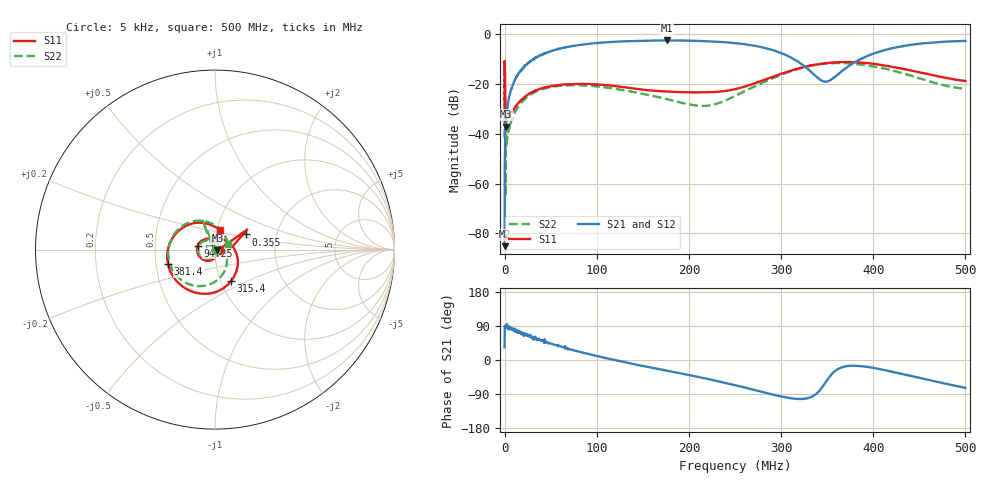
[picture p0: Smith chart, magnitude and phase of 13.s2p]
#  HZ  S  MA  R  50.00
! Rohde & Schwarz Vector Network Analyzer
! Rohde-Schwarz,ZNL6-2Port,1323001206101378,1.50.1.34-21.10.1.104
! Created: UTC 10/21/2024, 2:43:58 AM
! freq[Hz]  mag:S11  ang:S11  mag:S21  ang:S21  mag:S12  ang:S12  mag:S22  ang:S22
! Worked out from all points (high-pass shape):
!   10001 points, 5 kHz to 500 MHz, reference 50 ohm
!   highest |S21| = -2.50 dB at 176.2 MHz (marker M1); lowest = -85.2 dB at 5 kHz (marker M2)
!   |S21| within 3 dB of the highest: 62.95 MHz to 282.4 MHz (219.4 MHz wide, 127 % of centre); 422 MHz to end of sweep
!   lowest |S11| = -37.1 dB at 1.205 MHz (marker M3), VSWR 1.03, Z = 51.3 - j0.451 ohm
!   |S11| at or under -10 dB: start of sweep to end of sweep
!   |S22| runs from -65.2 to -10.9 dB; largest |S21 - S12| = 0.085
!   S11 on the Smith chart (normalised r, x): 5 kHz: 1.05, +0.00; 355 kHz: 1.39, +0.24; 94.25 MHz: 0.82, +0.04; 315.4 MHz: 1.12, -0.41; 381.4 MHz: 0.58, -0.10; 500 MHz: 1.03, +0.23
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5000  0.02251 1.1  5.509e-05 33.7  1.001e-05 114.1  0.008225 -27.2
354996.5  0.1909 26.2  0.003843 88.8  0.003578 89.5  0.1481 120.7
1204988  0.01399 -18.3  0.01339 87.4  0.01348 87.5  0.006824 -30.3
2654974  0.02098 -24.5  0.03108 92.9  0.02693 79.4  0.007904 -64.1
3104969  0.02034 -28.4  0.03431 84.2  0.03394 87.0  0.008835 -61.3
4454956  0.02193 -38.8  0.04942 82.4  0.048 86.6  0.01153 -70.3
9004910  0.02935 -64.7  0.09769 80.3  0.09743 79.4  0.02202 -90.2
1.585484e7  0.04326 -87.0  0.1695 73.7  0.1692 74.1  0.03734 -103.7
4.090459e7  0.08249 -134.2  0.392 50.6  0.3931 51.7  0.07853 -141.4
8.335417e7  0.1002 175.6  0.6162 20.4  0.6178 21.1  0.09401 173.4
9.425406e7  0.09946 166.9  0.6505 13.8  0.6525 14.7  0.09146 164.5
1.667033e8  0.07222 117.5  0.7486 -23.5  0.7516 -22.7  0.05453 110.9
1.762032e8  0.07057 111.2  0.7503 -28.1  0.7529 -27.3  0.04963 102.8
2.174028e8  0.06793 78.3  0.7271 -48.5  0.7284 -47.4  0.0362 47.1
2.500025e8  0.07874 37.1  0.6638 -66.3  0.6638 -64.9  0.0575 -13.1
3.154018e8  0.1969 -63.0  0.3047 -102.3  0.3052 -100.6  0.1944 -98.0
3.333517e8  0.2389 -90.5  0.1701 -96.9  0.1706 -95.1  0.2359 -123.0
3.502515e8  0.2651 -117.2  0.1126 -51.9  0.1129 -50.1  0.2588 -146.9
3.814012e8  0.2741 -163.0  0.2834 -15.1  0.2846 -13.3  0.2526 169.9
4.167008e8  0.2282 152.8  0.504 -28.9  0.503 -27.4  0.1952 125.2
4.524505e8  0.1682 117.1  0.6516 -48.5  0.6528 -47.2  0.1262 83.8
5e8  0.1148 76.7  0.7336 -73.6  0.7328 -72.6  0.07944 22.7
